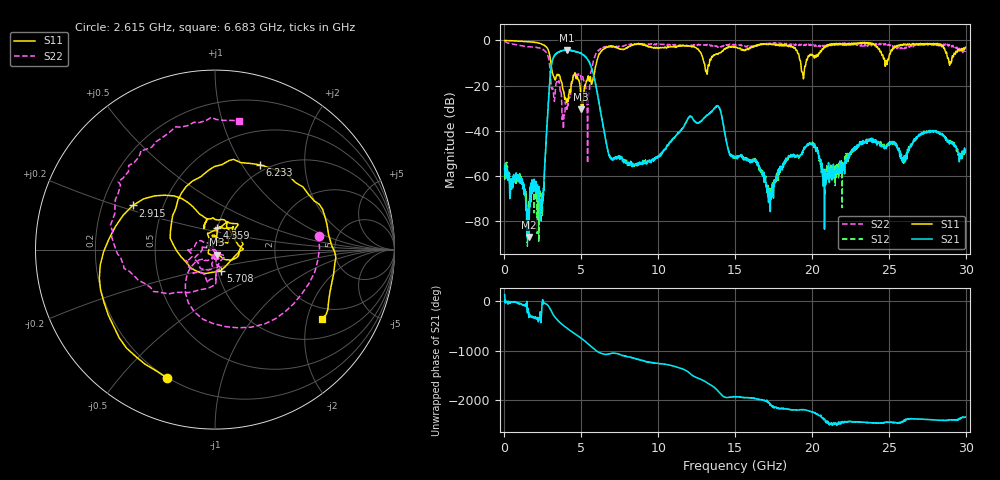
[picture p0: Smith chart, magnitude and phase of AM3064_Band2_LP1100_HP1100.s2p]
# Hz S DB R 50.0
!freq dBS11 angS11 dBS21 angS21 dBS12 angS12 dBS22 angS22
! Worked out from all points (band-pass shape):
!   1600 points, 10 MHz to 29.98 GHz, reference 50 ohm
!   highest |S21| = -4.24 dB at 4.059 GHz (marker M1); lowest = -87.0 dB at 1.603 GHz (marker M2)
!   |S21| within 3 dB of the highest: 3.214 GHz to 5.256 GHz (2.042 GHz wide, 48.2 % of centre)
!   lowest |S11| = -30.4 dB at 4.996 GHz (marker M3), VSWR 1.06, Z = 50.8 - j2.95 ohm
!   |S11| at or under -10 dB: 3.02 GHz to 5.988 GHz (2.968 GHz wide, 65.9 % of centre); 12.98 GHz to 13.33 GHz (348.6 MHz wide, 2.65 % of centre); 19.27 GHz to 19.61 GHz (338.9 MHz wide, 1.74 % of centre)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
!   |S22| runs from -54.3 to -0.3 dB; largest |S21 - S12| = 0.017
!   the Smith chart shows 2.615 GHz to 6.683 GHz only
!   S11 on the Smith chart (normalised r, x): 2.615 GHz: 0.20, -0.68; 2.915 GHz: 0.33, +0.23; 4.359 GHz: 0.99, +0.24; 5.708 GHz: 1.03, -0.24; 6.233 GHz: 0.91, +1.20; 6.683 GHz: 1.58, -2.46
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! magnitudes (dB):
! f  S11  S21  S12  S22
! 10 MHz  0.0  -56.6  -54.8  -0.3
! 1.603 GHz  -0.6  -87.0  -73.5  -2.8
! 2.409 GHz  -1.6  -75.8  -69.6  -3.7
! 2.615 GHz  -2.3  -55.9  -56.1  -4.7
! 2.915 GHz  -5.7  -20.8  -20.7  -9.6
! 3.215 GHz  -16.2  -7.2  -7.2  -26.0
! 4.059 GHz  -27.0  -4.2  -4.2  -30.5
! 4.359 GHz  -18.3  -4.6  -4.5  -19.2
! 4.996 GHz  -30.4  -5.9  -5.8  -17.4
! 5.015 GHz  -29.6  -5.9  -5.9  -17.4
! 5.408 GHz  -16.7  -8.4  -8.3  -54.3
! 5.708 GHz  -18.4  -13.0  -13.0  -11.6
! 6.233 GHz  -5.4  -30.8  -30.6  -3.6
! 6.683 GHz  -3.0  -47.4  -47.5  -2.7
! 10 GHz  -3.4  -51.3  -51.1  -1.8
! 13.82 GHz  -5.9  -28.9  -28.9  -2.5
! 15 GHz  -2.7  -51.9  -51.9  -1.8
! 17.25 GHz  -1.5  -67.2  -74.1  -1.2
! 19.99 GHz  -6.2  -46.0  -45.7  -1.8
! 20.85 GHz  -3.0  -57.4  -56.9  -2.5
! 25 GHz  -8.0  -46.2  -45.2  -1.8
! 29.98 GHz  -3.0  -48.7  -49.5  -4.7
